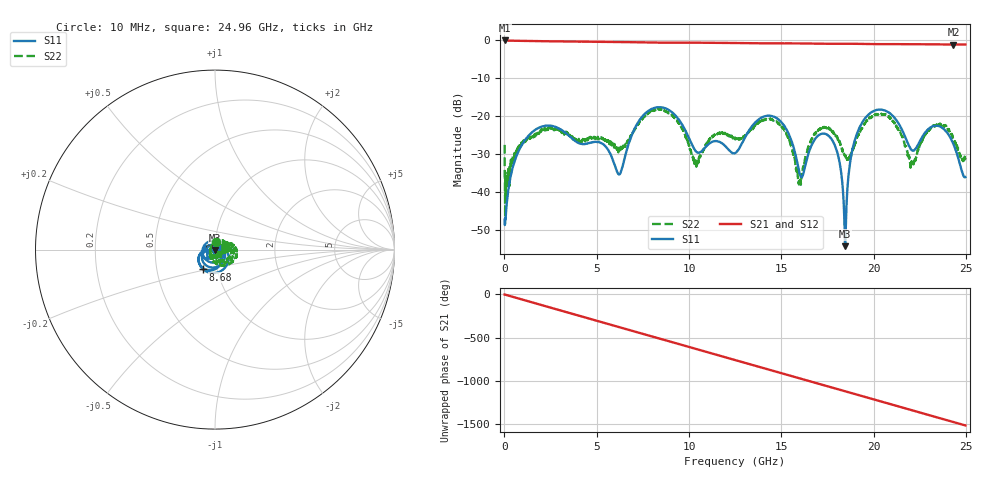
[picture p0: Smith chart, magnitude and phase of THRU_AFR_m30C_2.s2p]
!Keysight Technologies,M9372A,MY54321388,A.12.55.09
!Automatic Fixture Removal (AFR)
!Date: Wednesday, May 22, 2019 8:35:14 AM
!S2P File: Measurements: S11,S21,S12,S22:
# MHz S  RI  R 50
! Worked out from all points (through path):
!   2496 points, 10 MHz to 24.96 GHz, reference 50 ohm
!   highest |S21| = -0.01 dB at 40 MHz (marker M1); lowest = -1.1 dB at 24.31 GHz (marker M2)
!   group delay of S21, straight-line fit = 168 ps
!   lowest |S11| = -54.2 dB at 18.45 GHz (marker M3), VSWR 1.00, Z = 50 - j0.191 ohm
!   |S11| at or under -10 dB: start of sweep to end of sweep
!   |S22| runs from -46.5 to -17.9 dB; largest |S21 - S12| = 1.4e-15
!   S11 on the Smith chart (normalised r, x): 10 MHz: 1.01, +0.00; 8.68 GHz: 0.86, -0.19; 24.96 GHz: 1.03, +0.02
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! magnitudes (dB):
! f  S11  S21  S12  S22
! 10 MHz  -47.2  -0.1  -0.1  -27.5
! 40 MHz  -48.2  0.0  0.0  -46.5
! 540 MHz  -32.0  -0.1  -0.1  -29.7
! 1.44 GHz  -24.4  -0.2  -0.2  -25.6
! 4.17 GHz  -27.3  -0.3  -0.3  -26.7
! 6.23 GHz  -35.3  -0.4  -0.4  -28.5
! 8.33 GHz  -17.6  -0.6  -0.6  -18.1
! 8.68 GHz  -17.8  -0.6  -0.6  -18.6
! 10.34 GHz  -29.1  -0.6  -0.6  -32.6
! 12.49 GHz  -29.7  -0.7  -0.7  -25.7
! 14.53 GHz  -20.0  -0.8  -0.8  -21.0
! 16 GHz  -35.3  -0.8  -0.8  -36.8
! 16.65 GHz  -27.4  -0.8  -0.8  -25.9
! 17.83 GHz  -27.0  -0.9  -0.9  -24.6
! 18.45 GHz  -54.2  -0.9  -0.9  -30.5
! 18.76 GHz  -30.9  -0.9  -0.9  -29.9
! 19.18 GHz  -23.5  -0.9  -0.9  -24.9
! 20.81 GHz  -19.0  -1.0  -1.0  -20.1
! 22.06 GHz  -28.9  -1.0  -1.0  -32.1
! 23.17 GHz  -22.7  -1.0  -1.0  -22.8
! 24.31 GHz  -27.3  -1.1  -1.1  -26.3
! 24.96 GHz  -36.0  -1.1  -1.1  -30.9
